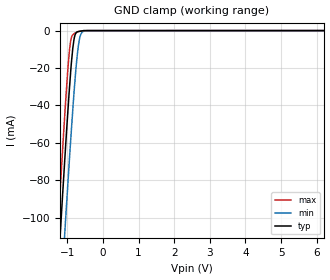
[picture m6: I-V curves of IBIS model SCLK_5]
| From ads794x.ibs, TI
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|   SCLK 5V Model
[Model] SCLK_5
Model_type   Input
Vinl = 1.5
Vinh = 3.5
|   typ   min   max
|   (Nom PVT)   (Fast PVT)  (Slow PVT)
C_comp   7.9207730e-13   6.6456320e-13  9.1956910e-13
|POWER = 5V
[Model Spec]
Vinl   1.5   1.35   1.65
Vinh   3.5   3.15   3.85
|Vinl = 0.3 X DVDD
|Vinh = 0.7 X DVDD
[Voltage Range]   5   4.75   5.25
[Temperature Range]   27   125   -40
[Power Clamp Reference]   5   4.75   5.25
[GND Clamp Reference]   0   0   0
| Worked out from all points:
|   GND clamp passes 1 mA (typ) near -0.74 V on its own axis
[GND Clamp]
|   Voltage   I(typ)   I(min)   I(max)
-5V       -1.409A    -1.433A    -1.396A
-1.296V   -140.7mA   -179.6mA   -116.9mA
-1.257V   -128.1mA   -167.2mA   -104.3mA
-1.194V   -107.9mA   -147mA     -83.76mA
-1.085V   -73.59mA   -112.8mA   -49.43mA
-1.047V   -61.81mA   -100.9mA   -38.07mA
-935.3mV  -29.91mA   -67.37mA   -9.922mA
-810.2mV  -4.597mA   -33.02mA   -1.71mA
-721.3mV  -642uA     -13.4mA    -812.8uA
-610.8mV  -260.5uA   -1.615mA   -227.9uA
-431.8mV  -16.09uA   -19.14uA   -15.55uA
9.985V    0A         0A         0A
[POWER Clamp]
|   SCR cell for ESD function. Effects occurr above VDD x 2
|   Voltage   I(typ)   I(min)   I(max)
-5V       0A         0A         0A
0V        0A         0A         0A
10V       0A         0A         0A
